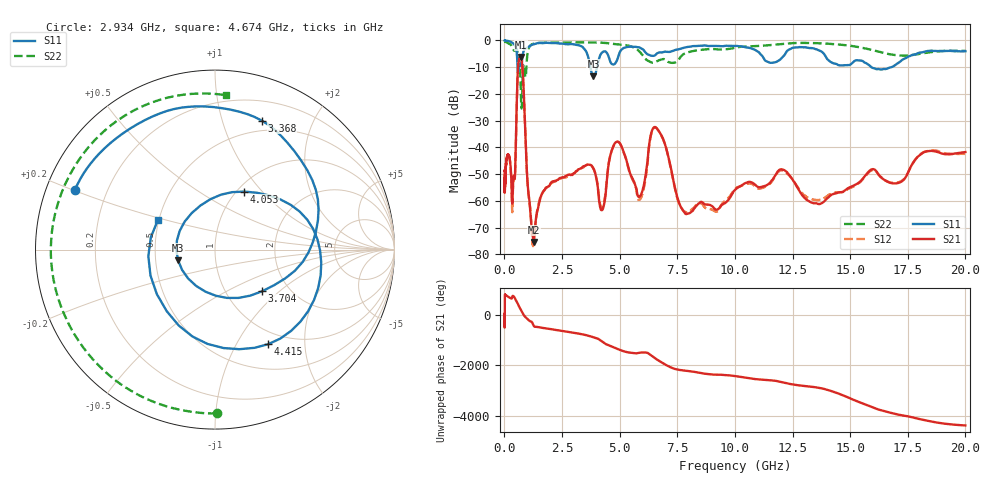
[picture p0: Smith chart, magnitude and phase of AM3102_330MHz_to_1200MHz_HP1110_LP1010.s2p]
! Date/Time: Tue, Sep 11, 2018 5:23 PM
! Network Analyzer: Agilent Technologies E8362B Rev: A.07.50.63
! Sweep from 0.010 to 20.000 GHz, 1601 Points, Sweep Type: LOG
! Power Supply: 4.949 V, 0.001 A
# Hz S DB R 50
!freq MagS11 AngS11 MagS21 AngS21 MagS12 AngS12 MagS22 AngS22
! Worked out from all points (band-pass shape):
!   1601 points, 10 MHz to 20 GHz, reference 50 ohm
!   highest |S21| = -6.21 dB at 702.3 MHz (marker M1); lowest = -75.4 dB at 1.266 GHz (marker M2)
!   |S21| within 3 dB of the highest: 599.9 MHz to 773.9 MHz (174 MHz wide, 25.3 % of centre)
!   lowest |S11| = -13.4 dB at 3.865 GHz (marker M3), VSWR 1.54, Z = 32.8 - j4.17 ohm
!   |S11| at or under -10 dB: 573.5 MHz to 626.2 MHz (52.7 MHz wide, 8.79 % of centre); 3.726 GHz to 4.021 GHz (295 MHz wide, 7.61 % of centre); 15.91 GHz to 16.8 GHz (883.7 MHz wide, 5.4 % of centre)
!   |S22| runs from -25.5 to -0.2 dB; largest |S21 - S12| = 0.0066
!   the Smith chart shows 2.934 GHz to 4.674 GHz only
!   S11 on the Smith chart (normalised r, x): 2.934 GHz: 0.08, +0.20; 3.368 GHz: 0.39, +1.35; 3.704 GHz: 1.47, -0.78; 4.053 GHz: 1.08, +0.80; 4.415 GHz: 0.82, -1.36; 4.674 GHz: 0.49, +0.19
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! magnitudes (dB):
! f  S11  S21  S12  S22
! 10 MHz  -0.1  -48.7  -49.9  -0.2
! 35.55 MHz  -0.1  -51.3  -50.1  -0.5
! 126.4 MHz  -0.2  -43.1  -43.4  -0.9
! 254.1 MHz  -0.5  -45.9  -45.9  -1.5
! 341.1 MHz  -1.0  -61.0  -64.1  -2.5
! 447.2 MHz  -1.8  -51.9  -51.5  -3.9
! 580.7 MHz  -11.1  -11.8  -11.8  -4.6
! 702.3 MHz  -9.2  -6.2  -6.2  -15.2
! 1.266 GHz  -1.5  -75.4  -76.3  -1.3
! 1.59 GHz  -1.0  -58.3  -58.1  -0.9
! 2.934 GHz  -1.4  -50.4  -50.1  -0.8
! 3.368 GHz  -2.3  -47.6  -47.8  -0.8
! 3.704 GHz  -9.1  -46.6  -46.3  -0.8
! 3.865 GHz  -13.4  -48.0  -47.9  -0.8
! 4.053 GHz  -8.8  -55.0  -54.6  -0.8
! 4.415 GHz  -4.4  -55.4  -54.7  -1.0
! 4.674 GHz  -8.9  -40.7  -40.8  -1.3
! 5.652 GHz  -2.4  -53.5  -53.8  -2.9
! 6.58 GHz  -5.2  -32.6  -32.7  -8.0
! 7.958 GHz  -2.5  -64.9  -64.4  -4.5
! 13.61 GHz  -3.7  -61.2  -59.7  -1.1
! 20 GHz  -4.1  -41.8  -42.4  -3.9
